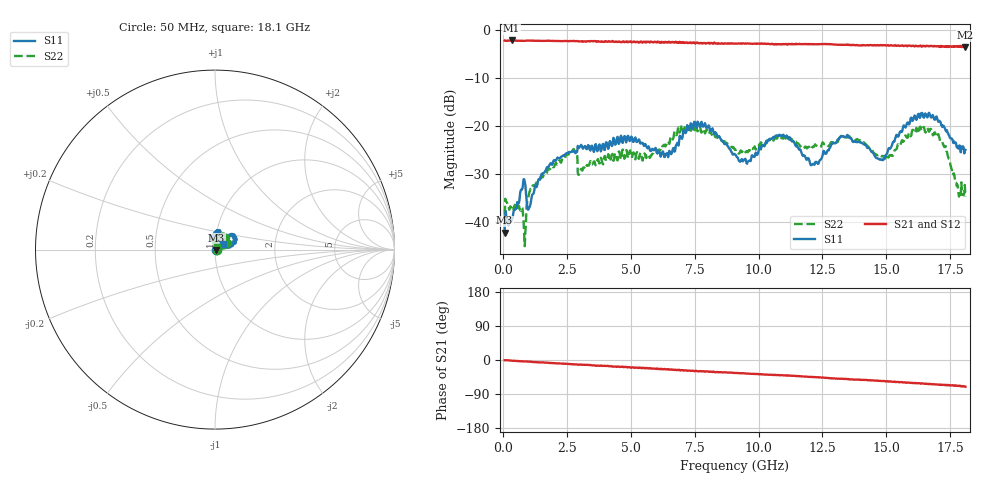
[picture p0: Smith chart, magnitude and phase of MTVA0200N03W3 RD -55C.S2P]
! Network Analyzer HP8720D.06.14 Serial No. US36140669
! 17 Jan 2005  11:58:46
! Frequency  S11  S21  S12  S22
# HZ  S  DB R 50
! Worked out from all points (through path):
!   801 points, 50 MHz to 18.1 GHz, reference 50 ohm
!   highest |S21| = -2.24 dB at 320.8 MHz (marker M1); lowest = -3.7 dB at 18.1 GHz (marker M2)
!   group delay of S21, straight-line fit = 10.3 ps
!   lowest |S11| = -42.3 dB at 50 MHz (marker M3), VSWR 1.02, Z = 50.7 - j0.31 ohm
!   |S11| at or under -10 dB: start of sweep to end of sweep
!   |S22| runs from -45.1 to -19.6 dB; largest |S21 - S12| = 0.022
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5e7  -42.26 -23.3  -2.26 -0.7  -2.31 -1.1  -41.06 -0.6
3.2075e8  -39.74 26.0  -2.24 -1.6  -2.24 -1.9  -36.98 2.9
8.17125e8  -31.14 31.4  -2.32 -3.6  -2.30 -3.9  -42.54 -49.2
1.020188e9  -37.01 48.2  -2.28 -4.2  -2.29 -4.7  -33.84 91.7
1.76475e9  -28.57 75.3  -2.28 -7.3  -2.31 -7.6  -28.86 84.0
2.689812e9  -25.42 77.1  -2.36 -11.1  -2.36 -11.3  -25.38 88.1
3.073375e9  -24.15 75.5  -2.42 -12.7  -2.40 -12.9  -29.22 98.9
4.946062e9  -23.19 76.5  -2.50 -18.9  -2.48 -19.8  -25.30 87.7
6.074188e9  -25.60 89.8  -2.60 -23.9  -2.60 -23.9  -25.22 83.2
7.563312e9  -20.37 80.5  -2.70 -29.3  -2.82 -30.5  -19.71 39.7
9.075e9  -25.96 106.4  -2.88 -34.1  -2.87 -34.3  -25.01 23.7
9.6165e9  -27.32 82.8  -2.90 -36.0  -2.88 -36.2  -25.14 24.1
1.088e10  -22.04 98.1  -3.07 -39.8  -3.00 -40.3  -22.58 23.6
1.209838e10  -28.11 80.8  -3.00 -44.9  -3.01 -45.1  -24.49 36.3
1.327162e10  -22.20 47.9  -3.16 -49.7  -3.15 -50.1  -22.12 43.5
1.476075e10  -27.07 42.1  -3.23 -54.8  -3.24 -55.5  -25.97 28.7
1.509919e10  -24.64 20.5  -3.29 -57.0  -3.18 -57.2  -26.45 36.5
1.604681e10  -18.85 23.6  -3.32 -60.6  -3.46 -60.9  -20.85 31.6
1.667856e10  -17.30 36.3  -3.48 -63.5  -3.37 -63.5  -21.25 21.5
1.724262e10  -19.97 46.9  -3.52 -65.7  -3.46 -66.8  -24.00 9.0
1.780669e10  -24.46 47.7  -3.54 -68.6  -3.51 -69.3  -32.94 24.8
1.81e10  -25.02 37.0  -3.68 -70.5  -3.62 -71.4  -34.77 41.2
